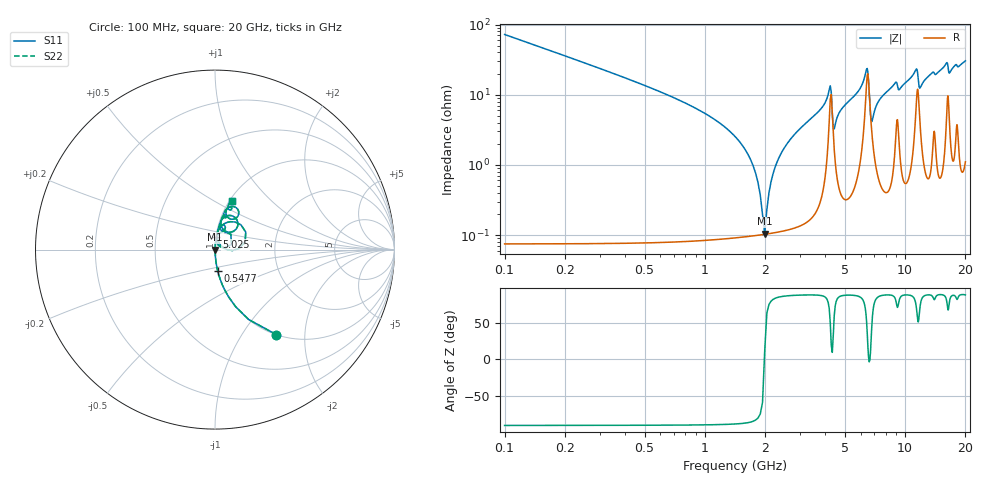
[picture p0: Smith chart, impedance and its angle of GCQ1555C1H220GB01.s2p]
!Murata Part Number: GCQ1555C1H220GB01
!These Parameters are Measured in Series Mode Connection
!Data Generated on Mar 13, 2026
!  o--ll--o
!Port1  Port2
!  o------o
!Operation Temp=25[degC], DC Bias Voltage=0[V]
!Freq. Start=100[MHz] Stop=20[GHz] 401[Steps]
# Hz S RI R 50
!Freq.(Hz) S11(Real) S11(Imag) S21(Real) S21(Imag) S12(Real) S12(Imag) S22(Real) S22(Imag)
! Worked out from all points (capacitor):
!   401 points, 100 MHz to 20 GHz, reference 50 ohm
!   read as one part in series: C = 22 pF near 199.5 MHz
!   lowest |Z| = 105 mohm at 1.99 GHz (marker M1)
!   series resonance near 1.985 GHz, so ESL is about 290 pH
!   S11 on the Smith chart (normalised r, x): 100 MHz: 1.00, -1.44; 547.8 MHz: 1.00, -0.24; 5.025 GHz: 1.01, +0.14; 20 GHz: 1.02, +0.61
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1e8  0.3426 -0.4741  0.6574 0.4741  0.6574 0.4741  0.3426 -0.4741
5.4775e8  0.0154 -0.1202  0.9846 0.1202  0.9846 0.1202  0.0154 -0.1202
1.54275e9  0.00128 -0.0187  0.9987 0.0187  0.9987 0.0187  0.00128 -0.0187
1.74175e9  0.00107 -0.00966  0.9989 0.00966  0.9989 0.00966  0.00107 -0.00966
1.891e9  0.00102 -0.00358  0.999 0.00358  0.999 0.00358  0.00102 -0.00358
1.9905e9  0.00102 0.000223  0.999 -0.000223  0.999 -0.000223  0.00102 0.000223
2.23925e9  0.00116 0.00906  0.9988 -0.00906  0.9988 -0.00906  0.00116 0.00906
2.43825e9  0.00138 0.0156  0.9986 -0.0156  0.9986 -0.0156  0.00138 0.0156
3.43325e9  0.00399 0.047  0.996 -0.047  0.996 -0.047  0.00399 0.047
4.1795e9  0.051 0.1004  0.949 -0.1004  0.949 -0.1004  0.051 0.1004
4.42825e9  0.0168 0.0273  0.9832 -0.0273  0.9832 -0.0273  0.0168 0.0273
5.02525e9  0.00828 0.0711  0.9917 -0.0711  0.9917 -0.0711  0.00828 0.0711
6.41825e9  0.1454 0.1371  0.8546 -0.1371  0.8546 -0.1371  0.1454 0.1371
6.7665e9  0.0373 0.0183  0.9627 -0.0183  0.9627 -0.0183  0.0373 0.0183
7.9605e9  0.0148 0.1031  0.9852 -0.1031  0.9852 -0.1031  0.0148 0.1031
1.005e10  0.0266 0.1437  0.9734 -0.1437  0.9734 -0.1437  0.0266 0.1437
1.13435e10  0.0997 0.1864  0.9003 -0.1864  0.9003 -0.1864  0.0997 0.1864
1.1841e10  0.054 0.1051  0.946 -0.1051  0.946 -0.1051  0.054 0.1051
1.338325e10  0.0431 0.1845  0.9569 -0.1845  0.9569 -0.1845  0.0431 0.1845
1.61195e10  0.1111 0.2375  0.8889 -0.2375  0.8889 -0.2375  0.1111 0.2375
1.67165e10  0.0673 0.185  0.9327 -0.185  0.9327 -0.185  0.0673 0.185
2e10  0.0926 0.2722  0.9074 -0.2722  0.9074 -0.2722  0.0926 0.2722
